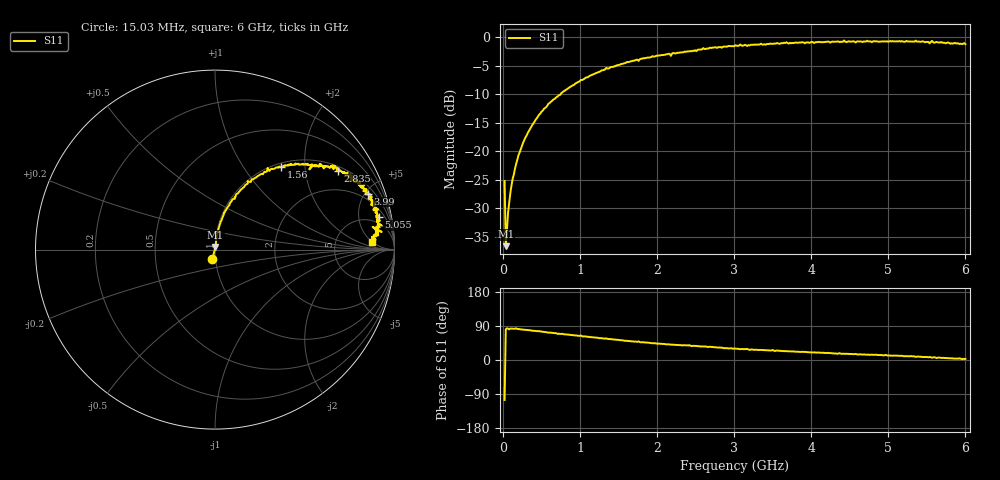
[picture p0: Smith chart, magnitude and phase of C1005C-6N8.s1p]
!	Network	Analyzer	HP8753E.07.74:	Oct	30	2002	Serial	No.	JP38451487
!	Hewlett-Packard
!	7	Sep	2009	8:29:48
!	Frequency	S11
#	HZ	S	RI	R	50
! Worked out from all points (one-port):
!   400 points, 15.03 MHz to 6 GHz, reference 50 ohm
!   lowest |S11| = -36.7 dB at 30.03 MHz (marker M1), VSWR 1.03, Z = 50.2 + j1.46 ohm
!   |S11| at or under -10 dB: start of sweep to 740.5 MHz
!   S11 on the Smith chart (normalised r, x): 15.03 MHz: 0.97, -0.10; 1.56 GHz: 1.06, +1.51; 2.835 GHz: 1.16, +2.99; 3.99 GHz: 1.49, +5.22; 5.055 GHz: 3.34, +8.87; 6 GHz: 13, +5
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1.502992e7  -0.0147 -0.0529
3.002985e7  0.00231 0.0145
6.00297e7  0.00361 0.0289
9.002955e7  0.0053 0.043
1.200294e8  0.00738 0.057
1.95029e8  0.0131 0.0914
2.850286e8  0.0235 0.13
4.650277e8  0.0496 0.205
7.650262e8  0.118 0.308
1.335023e9  0.293 0.455
1.515022e9  0.353 0.457
1.560022e9  0.369 0.462
2.265019e9  0.564 0.471
2.835016e9  0.683 0.439
3.015015e9  0.739 0.43
3.195014e9  0.761 0.381
3.495013e9  0.787 0.39
3.765011e9  0.823 0.345
3.99001e9  0.851 0.312
4.515007e9  0.883 0.252
5.055005e9  0.911 0.182
5.265004e9  0.91 0.157
5.355003e9  0.929 0.134
5.535002e9  0.878 0.126
5.565002e9  0.929 0.099
5.595002e9  0.89 0.116
5.625002e9  0.91 0.0796
6e9  0.873 0.0429
